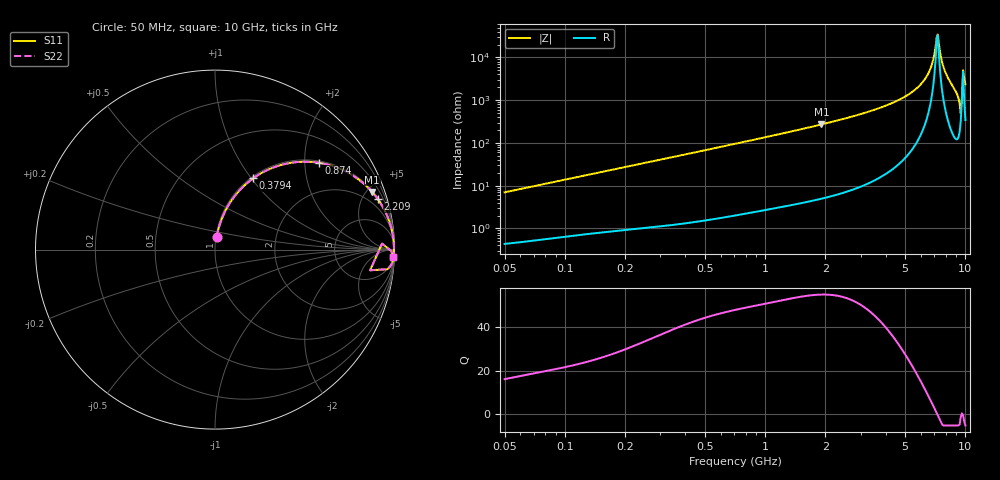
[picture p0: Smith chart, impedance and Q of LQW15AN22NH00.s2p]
!Murata Part Number: LQW15AN22NH00
!These Parameters are Measured in Series Mode Connection
!  o--[Z]--o
!Port1  Port2
!  o-------o
!Freq. Start=50[MHz] Stop=10[GHz], 401[Steps]
# Hz S RI R 50
!Freq.(Hz)	S 11(Real)	S 11(Imag)	S 21(Real)	S 21(Imag)	S 12(Real)	S 12(Imag)	S 22(Real)	S 22(Imag)
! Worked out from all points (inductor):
!   401 points, 50 MHz to 10 GHz, reference 50 ohm
!   read as one part in series: L = 22.1 nH near 51.34 MHz
!   highest Q = 54.7 at 1.91 GHz (marker M1), where L = 22.5 nH
!   self-resonance near 7.181 GHz
!   S11 on the Smith chart (normalised r, x): 50 MHz: 1.01, +0.14; 379.4 MHz: 1.03, +1.02; 874 MHz: 1.05, +2.36; 2.209 GHz: 1.12, +6.40; 10 GHz: 8, -46
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5e7  0.00908 0.0688  0.9909 -0.0688  0.9909 -0.0688  0.00908 0.0688
1.214486e8  0.0334 0.1595  0.9666 -0.1595  0.9666 -0.1595  0.0334 0.1595
2.949953e8  0.1437 0.3372  0.8563 -0.3372  0.8563 -0.3372  0.1437 0.3372
3.794145e8  0.2131 0.3972  0.7869 -0.3972  0.7869 -0.3972  0.2131 0.3972
7.071068e8  0.4766 0.4891  0.5234 -0.4891  0.5234 -0.4891  0.4766 0.4891
8.740297e8  0.5809 0.4834  0.4191 -0.4834  0.4191 -0.4834  0.5809 0.4834
1.717543e9  0.8478 0.3502  0.1522 -0.3502  0.1522 -0.3502  0.8478 0.3502
1.909537e9  0.8753 0.3214  0.1247 -0.3214  0.1247 -0.3214  0.8753 0.3214
2.209055e9  0.9069 0.2815  0.0931 -0.2815  0.0931 -0.2815  0.9069 0.2815
4.171863e9  0.9817 0.1213  0.0183 -0.1213  0.0183 -0.1213  0.9817 0.1213
5.225452e9  0.9919 0.0714  0.00806 -0.0714  0.00806 -0.0714  0.9919 0.0714
6.125686e9  0.9958 0.0371  0.00416 -0.0371  0.00416 -0.0371  0.9958 0.0371
6.632392e9  0.9969 0.0198  0.00314 -0.0198  0.00314 -0.0198  0.9969 0.0198
6.901252e9  0.9971 0.0111  0.00287 -0.0111  0.00287 -0.0111  0.9971 0.0111
7.086521e9  0.9972 0.00517  0.00277 -0.00517  0.00277 -0.00517  0.9972 0.00517
7.276762e9  0.9972 -0.00084  0.00276 0.00084  0.00276 0.00084  0.9972 -0.00084
7.37379e9  0.9972 -0.00388  0.00278 0.00388  0.00278 0.00388  0.9972 -0.00388
7.878683e9  0.9967 -0.0197  0.00325 0.0197  0.00325 0.0197  0.9967 -0.0197
8.994549e9  0.9908 -0.0638  0.00921 0.0638  0.00921 0.0638  0.9908 -0.0638
9.236013e9  0.9817 -0.0861  0.0183 0.0861  0.0183 0.0861  0.9817 -0.0861
9.359165e9  0.9627 -0.1091  0.0373 0.1091  0.0373 0.1091  0.9627 -0.1091
1e10  0.992 -0.0416  0.00798 0.0416  0.00798 0.0416  0.992 -0.0416
